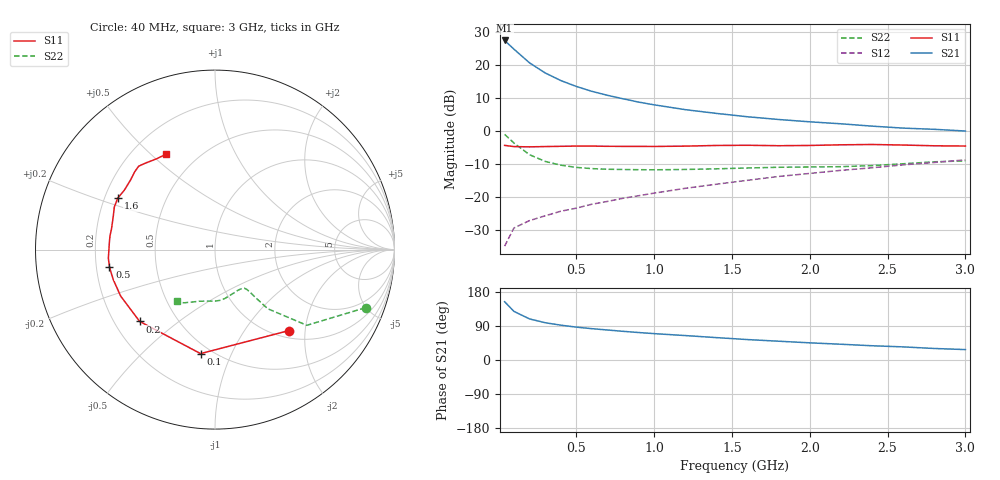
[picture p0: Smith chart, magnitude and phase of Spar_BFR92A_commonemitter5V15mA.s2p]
! Filename:  BFR92AD.S2P  Version:  2.0
! NXP part #: BFR92A  Date: May 1990
! Bias condition: Vce=5V, Ic=15mA
#  MHz  S  MA  R  50
! Freq  S11  S21  S12  S22  !GUM [dB]
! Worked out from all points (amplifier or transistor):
!   21 points, 40 MHz to 3 GHz, reference 50 ohm
!   highest |S21| = 27.6 dB at 40 MHz (marker M1)
!   |S21| within 3 dB of that: start of sweep to 108.5 MHz
!   unconditionally stable (mu >= 1): 699.9 MHz to 1.736 GHz
!   at 300 MHz: K = 0.72, MSG = 21.7 dB, |S12| = -25.7 dB
!   at 1 GHz: K = 1.06, MAG = 11.9 dB, |S12| = -18.8 dB
!   at 3 GHz: K = 0.98, MSG = 4.4 dB, |S12| = -8.7 dB
!   S11 on the Smith chart (normalised r, x): 40 MHz: 1.14, -1.64; 100 MHz: 0.44, -0.77; 200 MHz: 0.30, -0.37; 500 MHz: 0.25, -0.08; 1.6 GHz: 0.25, +0.23; 3 GHz: 0.34, +0.56
40  0.611 -47.6  23.94 153.8  0.018 70.1  0.899 -21.1
100  0.585 -97.9  17.65 128.3  0.034 53.6  0.663 -39.5
200  0.58 -136.4  10.94 108.4  0.044 49.3  0.441 -48.3
300  0.586 -153.8  7.705 98.4  0.052 50.8  0.349 -49.8
400  0.591 -163.6  5.905 92.0  0.061 54.1  0.306 -50.6
500  0.596 -170.5  4.8 86.8  0.068 57.6  0.283 -51.4
600  0.596 -175.5  4.045 82.7  0.078 60.2  0.271 -52.7
700  0.591 -179.8  3.519 79.2  0.086 62.2  0.265 -54.4
800  0.59 176.4  3.119 75.7  0.096 64.2  0.263 -56.3
900  0.59 172.5  2.777 72.5  0.105 65.3  0.261 -58.4
1000  0.588 168.7  2.522 69.6  0.115 66.6  0.26 -60.9
1200  0.595 162.6  2.131 64.5  0.136 68.3  0.263 -66.0
1400  0.609 157.1  1.869 59.1  0.157 68.8  0.269 -72.4
1600  0.613 152.1  1.661 53.9  0.18 69.8  0.277 -78.0
1800  0.604 146.7  1.51 49.6  0.206 69.4  0.284 -83.8
2000  0.609 140.9  1.392 45.3  0.229 69.5  0.287 -90.0
2200  0.623 135.9  1.299 41.6  0.255 68.7  0.29 -98.3
2400  0.63 132.4  1.197 37.6  0.279 68.7  0.301 -107.1
2600  0.618 128.7  1.117 34.6  0.309 67.3  0.321 -114.3
2800  0.602 123.0  1.071 30.4  0.336 65.4  0.344 -120.4
3000  0.597 117.1  1.009 27.5  0.368 64.8  0.355 -126.1
